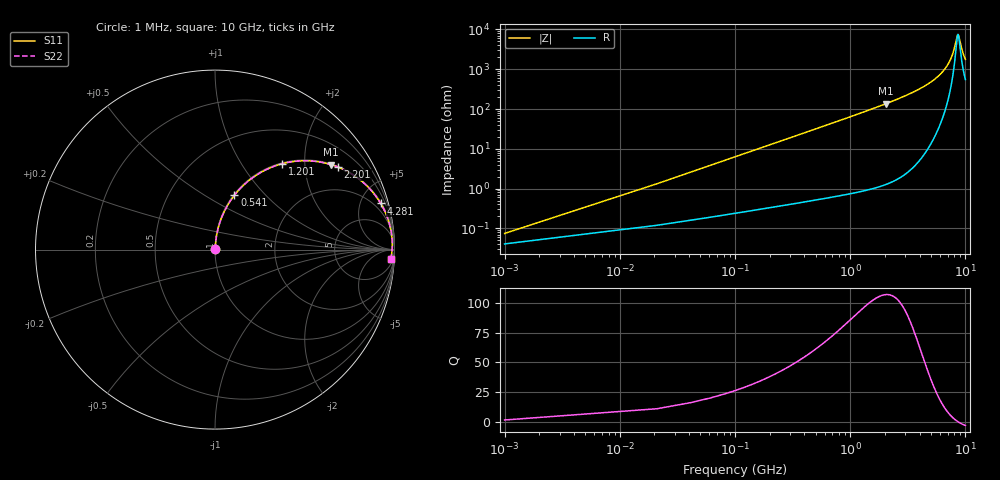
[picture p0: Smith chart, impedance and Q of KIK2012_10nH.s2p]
!version-2
!date-01.2022
!Series
# MHz S RI R 50
!Freq ReS11 ImS11 ReS21 ImS21 ReS12 ImS12 ReS22 ImS22
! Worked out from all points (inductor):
!   501 points, 1 MHz to 10 GHz, reference 50 ohm
!   read as one part in series: L = 10 nH near 41 MHz
!   highest Q = 107 at 2.041 GHz (marker M1), where L = 10.6 nH
!   self-resonance near 8.64 GHz
!   S11 on the Smith chart (normalised r, x): 1 MHz: 1.00, +0.00; 541 MHz: 1.01, +0.68; 1.201 GHz: 1.02, +1.54; 2.201 GHz: 1.03, +2.96; 4.281 GHz: 1.13, +7.14; 10 GHz: 12, -34
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1  0.000409 0.000628  0.9996 -0.000628  0.9996 -0.000628  0.000409 0.000628
61  0.00337 0.0381  0.9966 -0.0381  0.9966 -0.0381  0.00337 0.0381
81  0.00474 0.0505  0.9953 -0.0505  0.9953 -0.0505  0.00474 0.0505
121  0.00831 0.0752  0.9917 -0.0752  0.9917 -0.0752  0.00831 0.0752
181  0.0158 0.1116  0.9842 -0.1116  0.9842 -0.1116  0.0158 0.1116
281  0.0338 0.1701  0.9662 -0.1701  0.9662 -0.1701  0.0338 0.1701
541  0.1081 0.3027  0.8919 -0.3027  0.8919 -0.3027  0.1081 0.3027
821  0.2162 0.4053  0.7838 -0.4053  0.7838 -0.4053  0.2162 0.4053
1201  0.3733 0.4783  0.6267 -0.4783  0.6267 -0.4783  0.3733 0.4783
1681  0.5462 0.4931  0.4538 -0.4931  0.4538 -0.4931  0.5462 0.4931
2041  0.6473 0.4732  0.3527 -0.4732  0.3527 -0.4732  0.6473 0.4732
2201  0.6848 0.4599  0.3152 -0.4599  0.3152 -0.4599  0.6848 0.4599
3341  0.8562 0.345  0.1438 -0.345  0.1438 -0.345  0.8562 0.345
4281  0.9232 0.2573  0.0768 -0.2573  0.0768 -0.2573  0.9232 0.2573
5001  0.9522 0.2  0.0478 -0.2  0.0478 -0.2  0.9522 0.2
6681  0.9826 0.093  0.0174 -0.093  0.0174 -0.093  0.9826 0.093
7641  0.9873 0.0442  0.0127 -0.0442  0.0127 -0.0442  0.9873 0.0442
8341  0.9874 0.0126  0.0126 -0.0126  0.0126 -0.0126  0.9874 0.0126
8541  0.987 0.00412  0.013 -0.00412  0.013 -0.00412  0.987 0.00412
8701  0.9866 -0.0025  0.0134 0.0025  0.0134 0.0025  0.9866 -0.0025
9381  0.9837 -0.0292  0.0163 0.0292  0.0163 0.0292  0.9837 -0.0292
10000  0.98 -0.0517  0.02 0.0517  0.02 0.0517  0.98 -0.0517
